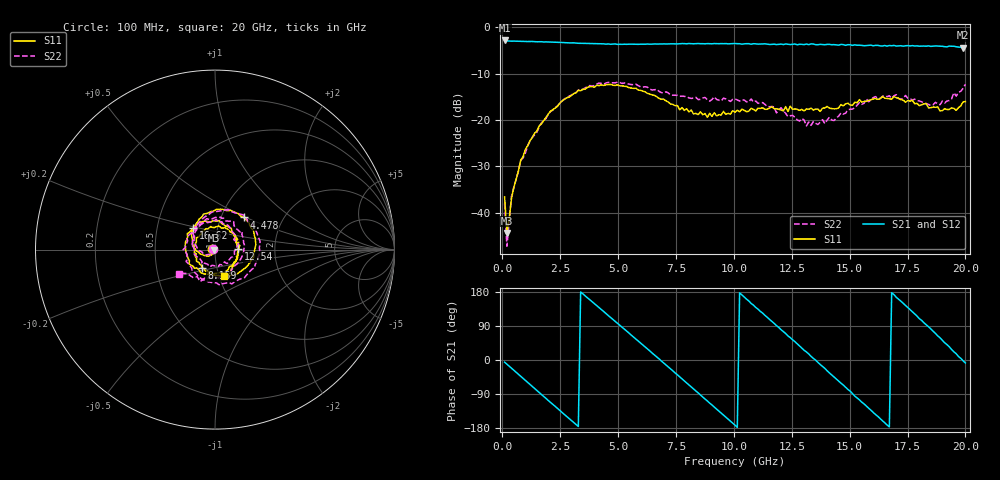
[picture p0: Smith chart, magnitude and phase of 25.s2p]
!Agilent Technologies,N5230C,MY49001569,A.09.33.09
!Agilent N5230C: A.09.33.09
!Date: Wednesday, July 29, 2015 14:52:45
!Correction: S11(Full 2 Port(1,2))
!S21(Full 2 Port(1,2))
!S12(Full 2 Port(1,2))
!S22(Full 2 Port(1,2))
!S2P File: Measurements: S11, S21, S12, S22:
# Hz S  dB  R 50
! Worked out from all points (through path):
!   201 points, 100 MHz to 20 GHz, reference 50 ohm
!   highest |S21| = -2.87 dB at 100 MHz (marker M1); lowest = -4.4 dB at 19.9 GHz (marker M2)
!   group delay of S21, straight-line fit = 150 ps
!   lowest |S11| = -44.4 dB at 199.5 MHz (marker M3), VSWR 1.01, Z = 49.5 - j0.247 ohm
!   |S11| at or under -10 dB: start of sweep to end of sweep
!   |S22| runs from -47.3 to -11.9 dB; largest |S21 - S12| = 0.029
!   S11 on the Smith chart (normalised r, x): 100 MHz: 0.97, +0.00; 4.478 GHz: 1.28, +0.48; 8.159 GHz: 0.84, -0.18; 12.54 GHz: 1.30, +0.01; 16.62 GHz: 0.77, +0.19; 20 GHz: 1.06, -0.32
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1e8  -36.65 170.1  -2.87 -5.7  -2.91 -6.1  -38.09 173.5
1.995e8  -44.40 -155.5  -2.98 -11.1  -3.00 -11.2  -47.26 -163.1
3.985e8  -36.88 -108.1  -3.02 -21.7  -3.01 -21.9  -36.48 -107.2
7.965e8  -28.70 -124.9  -3.05 -43.2  -3.05 -43.2  -28.74 -127.9
1.692e9  -20.87 -168.8  -3.14 -91.0  -3.19 -91.1  -20.63 -177.7
2.687e9  -15.54 138.4  -3.34 -144.1  -3.36 -144.1  -15.45 126.3
3.483e9  -13.44 96.5  -3.48 174.6  -3.49 174.2  -13.39 85.6
4.478e9  -12.42 48.4  -3.67 122.5  -3.61 122.1  -12.05 34.6
5.473e9  -13.05 1.8  -3.67 71.1  -3.71 70.4  -12.29 -11.0
6.7665e9  -15.35 -55.6  -3.63 3.2  -3.63 2.6  -13.84 -66.0
8.1595e9  -17.87 -126.0  -3.56 -70.9  -3.59 -71.8  -15.37 -129.7
8.9555e9  -18.61 -172.6  -3.57 -113.7  -3.58 -113.8  -15.98 -170.3
1.005e10  -18.34 121.3  -3.52 -171.9  -3.64 -172.9  -15.49 130.0
1.1443e10  -17.71 50.6  -3.67 112.6  -3.64 112.1  -17.12 47.3
1.25375e10  -17.73 1.1  -3.70 53.4  -3.88 52.9  -19.03 -13.8
1.3433e10  -17.89 -40.1  -3.63 4.3  -3.80 3.9  -20.37 -77.7
1.5025e10  -16.77 -125.9  -3.80 -82.2  -3.80 -83.4  -17.72 172.5
1.6617e10  -15.39 134.8  -4.10 -171.6  -3.93 -171.8  -14.99 77.8
1.67165e10  -15.46 134.5  -3.95 -176.4  -3.93 -177.8  -14.80 74.9
1.8408e10  -17.42 46.1  -4.03 87.8  -4.04 86.6  -16.67 -32.2
1.99005e10  -16.10 -56.2  -4.44 -2.1  -4.33 -4.1  -13.19 -142.9
2e10  -16.06 -70.4  -4.25 -7.8  -4.53 -9.7  -12.32 -145.8
